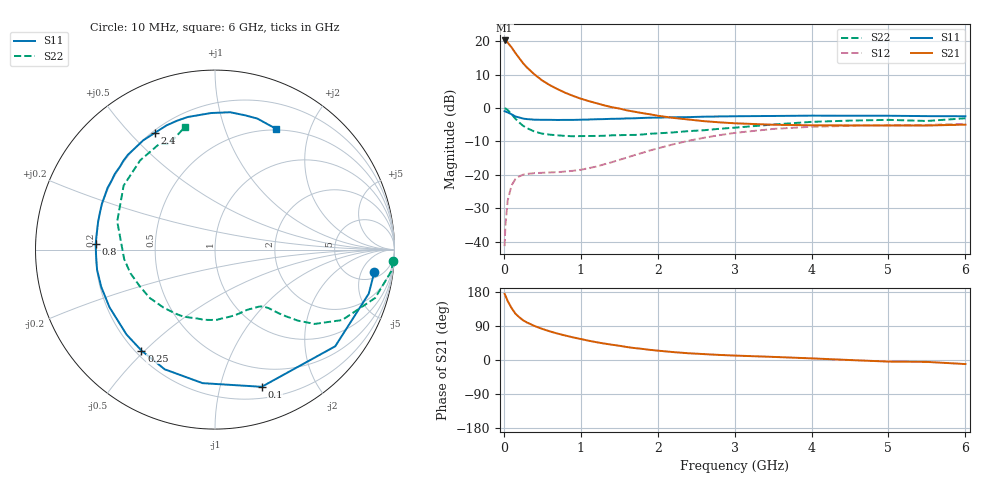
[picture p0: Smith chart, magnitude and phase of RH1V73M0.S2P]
! SIEMENS Small Signal Semiconductors
! BFR106
! Si NPN RF Bipolar Junction Transistor in SOT23
! VCE = 1.75 V  IC = 3 mA
! Common Emitter S-Parameters:  August  1996
# GHz  S  MA  R  50
!  f  S11  S21  S12  S22
! GHz  MAG  ANG  MAG  ANG  MAG  ANG  MAG  ANG
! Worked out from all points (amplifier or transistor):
!   36 points, 10 MHz to 6 GHz, reference 50 ohm
!   highest |S21| = 20.2 dB at 10 MHz (marker M1)
!   |S21| within 3 dB of that: start of sweep to 128.1 MHz
!   unconditionally stable (mu >= 1): 701.1 MHz to 2.267 GHz; 3.468 GHz to end of sweep
!   at 250 MHz: K = 0.40, MSG = 16.7 dB, |S12| = -19.9 dB
!   at 1.4 GHz: K = 1.24, MAG = 5.3 dB, |S12| = -16.2 dB
!   at 6 GHz: K = 1.02, MAG = -1.1 dB, |S12| = -4.7 dB
!   S11 on the Smith chart (normalised r, x): 10 MHz: 7, -9; 100 MHz: 0.31, -1.35; 250 MHz: 0.22, -0.49; 800 MHz: 0.20, +0.02; 2.4 GHz: 0.21, +0.59; 6 GHz: 0.48, +1.51
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0.01  0.8966 -8.0  10.25 174.4  0.0086 86.8  0.9948 -3.6
0.02  0.8911 -16.0  10.22 170.1  0.0173 80.4  0.9888 -7.1
0.05  0.8596 -38.8  9.528 155.5  0.0413 69.4  0.9322 -16.8
0.1  0.8075 -71.2  8.095 137.2  0.0698 54.5  0.8098 -29.0
0.15  0.7473 -95.3  6.665 122.5  0.0864 43.3  0.6929 -36.7
0.2  0.7235 -112.8  5.578 112.9  0.0952 37.1  0.6083 -40.6
0.25  0.6958 -126.1  4.686 104.8  0.1006 32.5  0.5429 -43.2
0.3  0.6832 -136.2  4.05 99.0  0.1033 30.1  0.5016 -45.0
0.4  0.6699 -151.4  3.172 89.7  0.1064 28.0  0.4438 -47.4
0.5  0.667 -161.8  2.58 82.0  0.1076 27.8  0.4142 -49.7
0.6  0.6666 -170.3  2.194 75.4  0.109 29.1  0.4001 -52.7
0.8  0.6655 177.3  1.69 64.5  0.1126 34.3  0.383 -60.2
1.1  0.6736 162.1  1.274 51.0  0.1259 44.9  0.382 -73.6
1.6  0.6998 142.8  0.923 34.2  0.1818 56.7  0.3958 -98.9
2.2  0.7283 123.3  0.713 20.9  0.2865 55.0  0.432 -131.6
2.4  0.7319 117.1  0.674 17.8  0.324 52.2  0.452 -143.3
3  0.7542 101.6  0.592 11.7  0.4248 40.6  0.5088 -174.0
3.5  0.7613 91.6  0.563 8.2  0.4872 30.1  0.567 163.9
4.5  0.7668 77.5  0.55 -0.1  0.5423 11.2  0.6491 129.9
5  0.7672 72.1  0.549 -4.2  0.5516 4.0  0.6658 117.7
5.5  0.7572 66.9  0.548 -5.0  0.559 0.6  0.6409 113.6
6  0.7541 63.4  0.565 -10.7  0.5805 -6.7  0.7032 103.8
